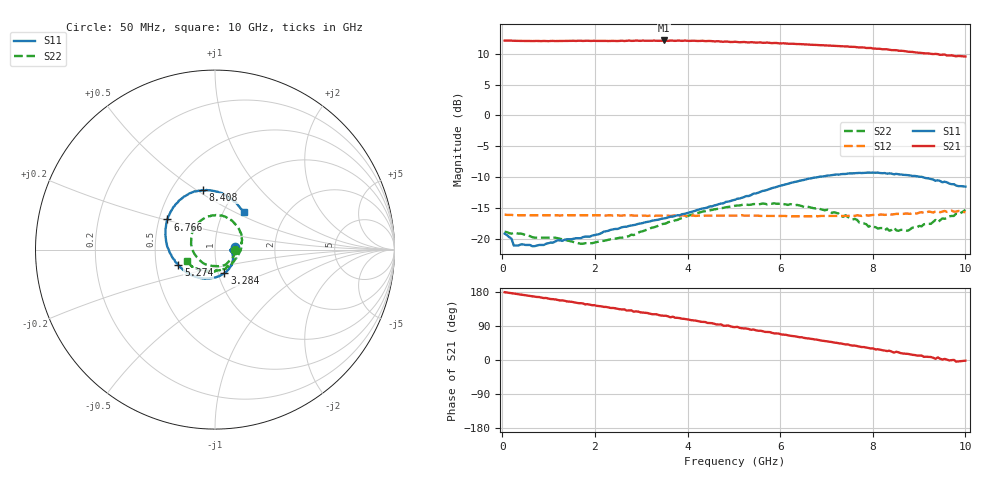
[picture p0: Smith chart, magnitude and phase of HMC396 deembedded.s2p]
!Hittite Microwave Corporation
!12 Elizabeth Drive
!Chelmsford, MA 01824
!Tel: 978-250-3343
!Fax: 978-250-3373
!Device: HMC396, DC-8 GHz InGaP HBT Gain Block MMIC Amplifier
!Misc: Vdd=+5V, Data includes (two) K connectors, Room
# MHZ S MA R 50
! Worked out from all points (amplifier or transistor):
!   201 points, 50 MHz to 10 GHz, reference 50 ohm
!   highest |S21| = 12.2 dB at 3.483 GHz (marker M1)
!   |S21| within 3 dB of that: start of sweep to end of sweep
!   unconditionally stable (mu >= 1): start of sweep to end of sweep
!   at 1.692 GHz: K = 1.10, MAG = 12.2 dB, |S12| = -16.2 dB
!   at 5.025 GHz: K = 1.06, MAG = 12.6 dB, |S12| = -16.2 dB
!   at 10 GHz: K = 1.13, MAG = 10.4 dB, |S12| = -15.7 dB
!   S11 on the Smith chart (normalised r, x): 50 MHz: 1.24, +0.04; 3.284 GHz: 1.07, -0.29; 5.274 GHz: 0.65, -0.12; 6.766 GHz: 0.55, +0.21; 8.408 GHz: 0.71, +0.53; 10 GHz: 1.24, +0.56
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50  0.11 8.2  4.043 179.0  0.157 0.2  0.114 -2.1
1741.5  0.103 -11.8  4.022 149.4  0.155 -9.8  0.091 -92.8
2686.75  0.125 -43.8  4.029 130.4  0.154 -14.9  0.104 -146.5
3283.75  0.141 -68.1  4.049 120.7  0.153 -19.2  0.124 -177.4
3383.25  0.143 -71.3  4.031 118.5  0.154 -20.5  0.128 177.8
3482.75  0.146 -76.6  4.059 116.8  0.153 -21.1  0.132 172.5
4328.5  0.176 -114.7  4.033 100.5  0.153 -25.3  0.166 135.9
5025  0.207 -145.2  3.962 86.8  0.154 -30.6  0.185 108.4
5273.75  0.222 -156.7  3.921 83.1  0.154 -30.7  0.189 99.9
5870.75  0.26 178.9  3.873 70.4  0.153 -34.3  0.194 79.2
6716.5  0.312 149.4  3.739 54.7  0.153 -38.7  0.177 45.0
6766.25  0.314 147.7  3.736 53.8  0.153 -38.9  0.176 43.4
7562.25  0.339 124.0  3.601 37.8  0.154 -42.4  0.143 1.1
8358.25  0.339 102.1  3.415 24.6  0.159 -44.5  0.116 -54.2
8408  0.337 101.3  3.389 21.9  0.157 -45.4  0.118 -57.3
9253.75  0.305 76.5  3.163 7.9  0.165 -50.8  0.132 -113.5
9353.25  0.295 74.3  3.157 3.1  0.166 -56.3  0.142 -122.8
9403  0.298 71.5  3.145 6.9  0.167 -49.9  0.136 -126.7
9502.5  0.287 68.2  3.114 1.3  0.166 -57.8  0.146 -126.5
9751.25  0.277 61.5  3.045 0.3  0.166 -53.6  0.153 -141.4
9801  0.27 58.1  3.02 -4.3  0.166 -57.5  0.16 -144.7
10000  0.265 52.6  3.008 -1.8  0.164 -52.3  0.171 -158.0
